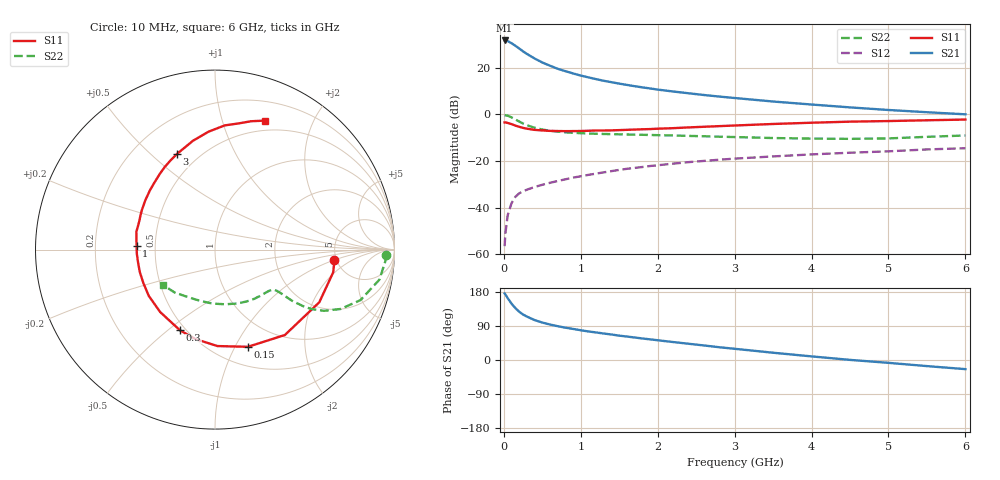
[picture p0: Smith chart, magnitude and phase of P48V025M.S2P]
! SIEMENS Small Signal Semiconductors
! BFP182
! Si NPN RF Bipolar Junction Transistor in SOT143
! VCE = 8 V  IC = 25 mA
! Common Emitter S-Parameters:  March  1996
# GHz  S  MA  R  50
!  f  S11  S21  S12  S22
! GHz  MAG  ANG  MAG  ANG  MAG  ANG  MAG  ANG
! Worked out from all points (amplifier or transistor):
!   36 points, 10 MHz to 6 GHz, reference 50 ohm
!   highest |S21| = 31.6 dB at 10 MHz (marker M1)
!   |S21| within 3 dB of that: start of sweep to 180.8 MHz
!   unconditionally stable (mu >= 1): 813.5 MHz to 5.601 GHz
!   at 250 MHz: K = 0.50, MSG = 30.0 dB, |S12| = -33.0 dB
!   at 1.4 GHz: K = 1.14, MAG = 16.7 dB, |S12| = -24.4 dB
!   at 6 GHz: K = 0.95, MSG = 7.3 dB, |S12| = -14.5 dB
!   S11 on the Smith chart (normalised r, x): 10 MHz: 4.80, -1.03; 150 MHz: 0.70, -1.13; 300 MHz: 0.47, -0.55; 1 GHz: 0.39, +0.02; 3 GHz: 0.38, +0.61; 6 GHz: 0.39, +1.38
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0.01  0.6681 -5.1  37.97 175.7  0.0015 84.9  0.9557 -1.7
0.02  0.6706 -10.9  37.91 173.1  0.0028 82.8  0.951 -4.0
0.05  0.651 -26.8  36.8 163.2  0.0069 83.0  0.9309 -10.4
0.1  0.6148 -50.7  33.12 148.8  0.0125 67.1  0.8575 -19.2
0.15  0.5718 -71.3  29.2 136.8  0.0171 60.8  0.774 -25.3
0.2  0.5375 -88.6  25.53 127.3  0.0203 57.5  0.6971 -29.3
0.25  0.5101 -102.3  22.15 120.0  0.0224 53.6  0.6332 -31.6
0.3  0.4902 -113.4  19.54 114.6  0.0243 52.8  0.5833 -32.7
0.4  0.463 -131.3  15.6 105.3  0.0277 51.6  0.5143 -33.6
0.5  0.4501 -145.1  12.8 98.8  0.0309 51.1  0.4705 -33.6
0.6  0.4404 -155.1  10.94 93.6  0.0341 52.1  0.4424 -33.5
0.7  0.4372 -163.4  9.406 89.2  0.0372 52.9  0.424 -33.6
0.8  0.4347 -170.8  8.351 85.3  0.0405 52.9  0.4105 -33.8
1  0.4376 177.1  6.72 78.5  0.047 53.8  0.3932 -34.8
1.1  0.4427 171.6  6.151 75.3  0.0504 53.6  0.3871 -35.6
1.5  0.4574 155.1  4.521 64.3  0.0644 53.0  0.3716 -40.0
2.2  0.5034 132.1  3.068 47.4  0.0876 48.5  0.3513 -51.2
3  0.5738 111.6  2.228 29.6  0.1121 41.4  0.325 -67.6
3.5  0.6189 101.4  1.872 19.2  0.1251 36.7  0.3096 -79.6
4.5  0.6941 85.5  1.402 0.3  0.1501 28.1  0.2973 -106.6
5.5  0.7429 74.3  1.105 -16.1  0.1765 20.2  0.3282 -133.3
6  0.7696 69.0  0.996 -24.1  0.1874 15.5  0.3512 -146.1
